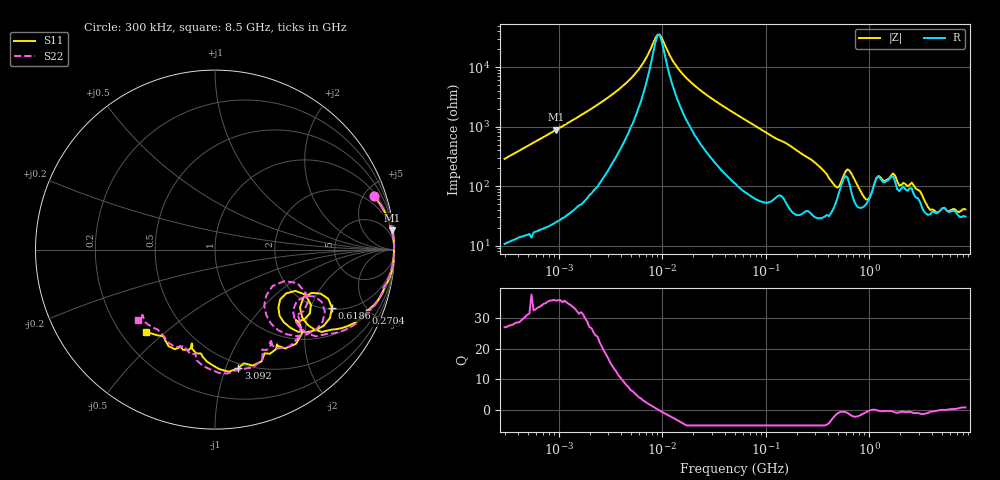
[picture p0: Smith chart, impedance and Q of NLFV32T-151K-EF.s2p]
! S-parameter Generated by TDK Corporation
! Copyright(C) 2015 TDK Corporation.
! All Rights Reserved.
! TDK P/N: NLFV32T-151K-EF (Inductors)
! Property: L=150uH at 796kHz
! Size(LxWxT): 3.2x2.5x2.2mm, 0.126x0.098x0.087inches
! Model Type: s2p (Touchstone File Format Version 1.0)
! Frequency: DC=Yes Start=0.3MHz Stop=8500MHz 225points Log-sweep
! Note:
! Model Generated on Jun. 23, 2015
! Hash(MD5):
! Port Assignments:
!  1 ---@@@--- 2
! Applicable Conditions:
!  Temperature = 25 degC
!  DC Bias Current = 0 A
!  Small Signal Operation
! Terms and conditions regarding TDK Simulation Models
! (1)This simulation model is being provided solely for informational purposes. Please refer to the specifications of the products in terms of detailed characteristics of such products.
! (2)In no event shall TDK Corporation of any of its subsidiaries be liable for any loss or damage arising, directly or indirectly,
!  From any information contained in this simulation model, including, but not limited to loss or damages arising from any inaccuracies, omissions or errors in connection with such information.
! (3)Any and all copyrights on this simulation model are owned by TDK Corporation.
!  Duplication or redistribution of this simulation model without prior written permission from TDK Corporation is prohibited.
! (4)This simulation model is subject to any modification or change without any prior notice.
! (5)Neither TDK Corporation nor any of its subsidiaries shall make any warranty, express or implied,
!  Including but not limited to the correctness, implied warranties of merchantability and fitness for a particular purpose with respect to this simulation models.
! (6)The use of this simulation model shall be deemed to have consented to the terms and conditions hereof.
# MHz S MA R 50
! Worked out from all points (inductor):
!   224 points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, 300 kHz to 8.5 GHz, reference 50 ohm
!   read as one part in series: L = 151 uH near 314.1 kHz
!   highest Q = 35.7 at 946.8 kHz (marker M1), where L = 149 uH
!   self-resonance near 9.007 MHz
!   S11 on the Smith chart (normalised r, x): 300 kHz: 1.25, +5.83; 270.4 MHz: 1.12, -4.69; 618.6 MHz: 2.08, -2.86; 3.092 GHz: 0.46, -1.11; 8.5 GHz: 0.30, -0.43
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0.3  0.9336 18.6  0.3251 -69.2  0.3293 -69.4  0.9328 18.7
0.9467989  0.9904 6.3  0.1118 -82.1  0.1123 -82.5  0.9908 6.2
1.72111  0.996 3.4  0.06079 -84.8  0.06099 -85.2  0.9967 3.3
4.954665  0.9975 0.8  0.01559 -80.5  0.0156 -80.9  0.9976 0.6
9.430415  0.9973 -0.2  0.002813 8.5  0.002806 8.3  0.9972 -0.4
16.37255  0.997 -1.1  0.01397 76.6  0.01398 76.3  0.9969 -1.3
51.67171  0.9952 -4.4  0.06137 81.6  0.0614 81.3  0.9922 -4.9
270.4017  0.9113 -22.9  0.3132 59.3  0.3134 59.1  0.9038 -24.6
283.1228  0.9055 -24.0  0.3291 58.3  0.3293 58.1  0.8974 -25.8
408.9767  0.751 -37.6  0.5172 38.4  0.5177 38.1  0.7412 -40.7
491.5417  0.5726 -34.2  0.549 16.4  0.5493 16.0  0.5512 -38.1
618.5683  0.7279 -26.4  0.3549 18.3  0.3551 18.1  0.7023 -29.4
743.4462  0.6877 -42.0  0.5166 23.6  0.5166 23.3  0.6622 -46.7
935.5712  0.4786 -42.4  0.6233 -0.5  0.6234 -1.1  0.4149 -48.7
1073.923  0.503 -27.2  0.5292 -18.5  0.5283 -18.7  0.4234 -24.5
1177.346  0.6161 -29.9  0.4035 -18.2  0.4032 -18.6  0.5616 -25.6
1551.304  0.6022 -41.4  0.3975 -15.1  0.3979 -15.7  0.6146 -39.9
1780.71  0.6921 -49.3  0.3722 -4.6  0.3723 -5.0  0.6814 -52.5
3091.568  0.6739 -78.9  0.4504 -18.4  0.4505 -18.5  0.6939 -84.3
3715.7  0.6243 -94.3  0.5425 -29.1  0.5439 -29.4  0.6267 -99.3
4895.91  0.5381 -103.8  0.5243 -53.3  0.5259 -54.4  0.563 -107.9
8500  0.5978 -129.8  0.3983 -101.1  0.3977 -100.4  0.5795 -137.6
